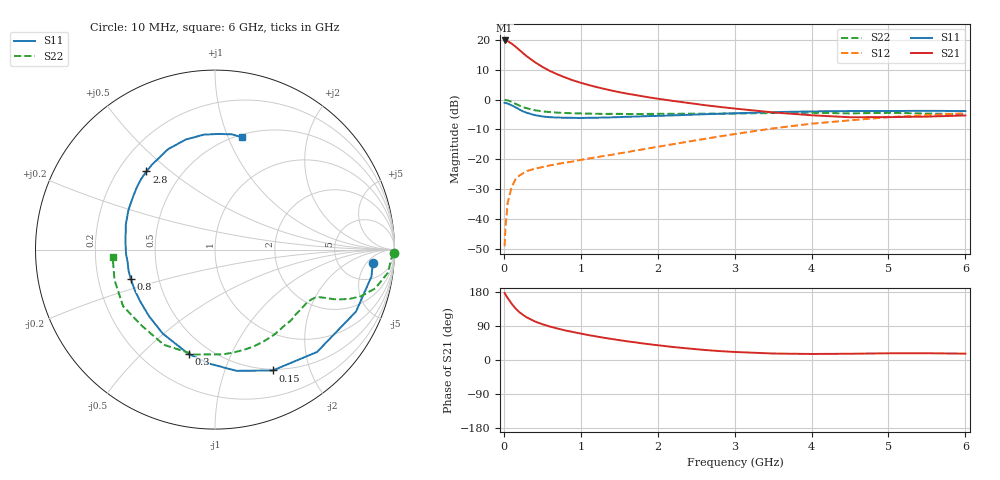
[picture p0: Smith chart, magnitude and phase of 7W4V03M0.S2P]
! Infineon Technologies  Discrete & RF Semiconductors
! BFS17W
! Si NPN RF Bipolar Junction Transistor in SOT323
! VCE = 4 V  IC = 3 mA
! Common Emitter S-Parameters:  August  1999
# GHz  S  MA  R  50
!  f  S11  S21  S12  S22
! GHz  MAG  ANG  MAG  ANG  MAG  ANG  MAG  ANG
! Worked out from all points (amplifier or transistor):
!   36 points, 10 MHz to 6 GHz, reference 50 ohm
!   highest |S21| = 19.8 dB at 10 MHz (marker M1)
!   |S21| within 3 dB of that: start of sweep to 194 MHz
!   unconditionally stable (mu >= 1): 712.1 MHz to 2.967 GHz; 4.191 GHz to end of sweep
!   at 250 MHz: K = 0.44, MSG = 20.1 dB, |S12| = -24.7 dB
!   at 1.4 GHz: K = 1.28, MAG = 7.6 dB, |S12| = -18.5 dB
!   at 6 GHz: K = 1.08, MAG = -2.1 dB, |S12| = -4.6 dB
!   S11 on the Smith chart (normalised r, x): 10 MHz: 11, -7; 150 MHz: 0.48, -1.47; 300 MHz: 0.39, -0.70; 800 MHz: 0.34, -0.15; 2.8 GHz: 0.32, +0.41; 6 GHz: 0.53, +1.13
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0.01  0.8827 -4.7  9.809 177.2  0.0035 85.1  0.9981 -1.1
0.02  0.8845 -9.8  9.801 173.4  0.0069 92.0  0.9831 -3.0
0.05  0.8582 -23.7  9.526 163.4  0.0187 78.6  0.9733 -7.5
0.1  0.8054 -45.1  8.72 149.0  0.0339 66.7  0.9186 -13.6
0.15  0.7462 -64.5  7.756 136.4  0.0457 58.6  0.8539 -17.7
0.2  0.6859 -80.0  6.841 126.6  0.0534 53.5  0.7971 -20.2
0.25  0.6358 -92.9  5.992 118.8  0.0583 49.2  0.7495 -21.7
0.3  0.6 -104.2  5.306 112.3  0.0636 47.3  0.7154 -22.7
0.4  0.5513 -121.8  4.272 102.1  0.0693 44.3  0.6647 -23.8
0.5  0.5222 -134.8  3.543 94.5  0.0742 44.0  0.6364 -24.6
0.6  0.507 -145.3  3.019 88.2  0.0791 45.2  0.6181 -25.7
0.8  0.4971 -160.7  2.344 78.0  0.0879 47.7  0.5963 -28.8
0.9  0.4955 -166.7  2.105 73.8  0.0922 49.4  0.5898 -30.5
1.1  0.4961 -177.1  1.761 65.7  0.1031 52.7  0.5828 -34.6
1.3  0.5013 174.3  1.521 58.7  0.1139 55.4  0.5765 -39.2
1.6  0.517 163.9  1.26 49.4  0.1318 59.2  0.5742 -46.4
2.2  0.5439 146.8  0.951 34.3  0.1793 64.6  0.5792 -62.6
2.8  0.5794 131.3  0.756 23.6  0.2409 65.4  0.5827 -80.1
3.5  0.6175 115.1  0.611 17.1  0.3298 61.8  0.5961 -101.3
4.5  0.6435 95.5  0.507 16.5  0.4496 50.0  0.5884 -134.0
5.5  0.649 81.6  0.519 17.8  0.5513 37.2  0.5851 -163.1
6  0.6438 76.3  0.543 16.8  0.5908 30.9  0.5717 -175.9
